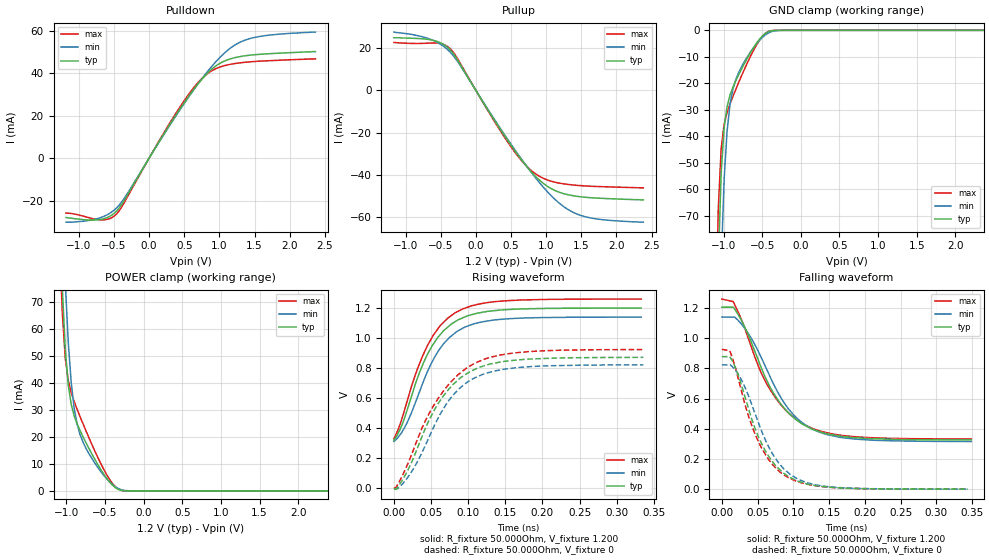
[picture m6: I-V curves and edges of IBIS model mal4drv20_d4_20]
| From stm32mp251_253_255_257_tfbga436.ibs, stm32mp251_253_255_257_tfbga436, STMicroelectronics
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[Model] mal4drv20_d4_20
Model_type   I/O
Polarity   Non-Inverting
Enable   Active-High
C_comp   1.838pF   1.835pF   1.848pF
C_comp_pullup   938.881fF   931.604fF   947.115fF
C_comp_pulldown 782.410fF   779.859fF   796.520fF
Vinh = 668.000mV
Vinl = 532.000mV
Vmeas = 600.000mV
Vref = 600.000mV
Rref = 50Ohms
Cref = 0pF
[Model Spec]
Vinh   668.000mV   638.000mV   698.000mV
Vinl   532.000mV   502.000mV   562.000mV
Vmeas   600.000mV   570.000mV   630.000mV
Vref   600.000mV   570.000mV   630.000mV
D_overshoot_ampl_h 0.24 NA   NA
D_overshoot_ampl_l 0.24 NA   NA
D_overshoot_area_l 300.000m NA   NA
D_overshoot_area_h 300.000m NA   NA
[Receiver Thresholds]
Vth = 600.000mV
Vth_min = 570.000mV
Vth_max = 630.000mV
Vinh_ac = 68.000mV
Vinh_dc = 68.000mV
Vinl_ac = -68.000mV
Vinl_dc = -68.000mV
Tslew_ac = 5.000ns
Threshold_sensitivity = 0.5
Reference_supply Pullup_ref
[Temperature Range]   25.000   125.000   -40.000
[Voltage Range]   1.200V   1.140V   1.260V
[GND Clamp Reference]   0.00V   0.00V   0.00V
[C Comp Corner]
| variable   typ   min   max
C_comp 1.848pF   1.838pF   1.835pF
C_comp_pullup 938.881fF   947.115fF   931.604fF
C_comp_pulldown 779.859fF   796.520fF   782.410fF
[Pulldown Reference]   0.00V   0.00V   0.00V
[POWER Clamp Reference]   1.200V   1.140V   1.260V
[Pullup Reference]   1.200V   1.140V   1.260V
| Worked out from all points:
|   slope of the pulldown table from 0 to 0.18 V, typ, clamps not added: 18.4 ohm
|   slope of the pullup table from 0 to 0.18 V, typ, clamps not added: 18.5 ohm
|   GND clamp passes 1 mA (typ) near -0.45 V on its own axis
|   POWER clamp passes 1 mA (typ) near -0.35 V on its own axis
|   rising waveform, R_fixture 50.000Ohm, V_fixture 1.200: 20-80 % time 46.3ps typ, 47.6ps min, 47ps max; typ from 0.321 V to 1.2 V
|   rising waveform, R_fixture 50.000Ohm, V_fixture 0: 20-80 % time 57.2ps typ, 56.6ps min, 62.2ps max; typ from -0.006 V to 0.872 V
|   falling waveform, R_fixture 50.000Ohm, V_fixture 1.200: 20-80 % time 57.7ps typ, 58.7ps min, 59.1ps max; typ from 1.21 V to 0.327 V
|   falling waveform, R_fixture 50.000Ohm, V_fixture 0: 20-80 % time 45.2ps typ, 47.2ps min, 44.8ps max; typ from 0.879 V to 0 V
[GND Clamp]
-1.184V   -365mA     -429.3mA   -336.5mA
-1.107V   -152.4mA   -215.7mA   -121.1mA
-1.069V   -88.87mA   -140.5mA   -67.62mA
-1.031V   -53.54mA   -88.39mA   -44.48mA
-992.7mV  -36.7mA    -56.18mA   -35.42mA
-954.6mV  -28.78mA   -37.93mA   -30.92mA
-916.4mV  -24.43mA   -27.89mA   -27.7mA
-840mV    -18.89mA   -18.42mA   -22.12mA
-763.6mV  -14.38mA   -13.51mA   -16.88mA
-572.7mV  -4.818mA   -5.067mA   -5.477mA
-458.2mV  -1.146mA   -1.695mA   -1.103mA
2.367V    25.44nA    625nA      8.401nA
[Power Clamp]
-1.167V   197.6mA    234.2mA    183.1mA
-1.091V   108mA      144mA      94.42mA
-1.053V   75.21mA    107.2mA    65.93mA
-1.015V   52.65mA    77.42mA    49.33mA
-976.4mV  39.37mA    55.31mA    41.02mA
-938.2mV  32.15mA    40.29mA    36.48mA
-900mV    27.91mA    30.75mA    33.22mA
-823.6mV  22.42mA    20.91mA    27.62mA
-632.7mV  11.76mA    10.36mA    14.83mA
-365.4mV  1.178mA    1.496mA    1.508mA
-212.7mV  14.35uA    76.22uA    9.056uA
2.384V    -16.74nA   -562.7nA   -5.86nA
[Pulldown]
-1.184V   -28mA      -30.2mA    -25.9mA
-725.5mV  -29.07mA   -28.41mA   -29mA
-572.7mV  -27.67mA   -26.26mA   -28.66mA
-458.2mV  -24.75mA   -23.28mA   -26.13mA
-343.6mV  -19.28mA   -18.42mA   -20.31mA
458.2mV   24.11mA    23.68mA    25.02mA
687.3mV   34.55mA    34.52mA    35.24mA
878.2mV   41.46mA    42.63mA    40.85mA
1.145V    46.59mA    51.48mA    44.06mA
1.375V    48.18mA    55.64mA    45.11mA
1.718V    49.14mA    57.9mA     45.84mA
2.367V    50.1mA     59.3mA     46.7mA
[Pullup]
-1.167V   25mA       27.69mA    22.76mA
-632.7mV  23.95mA    24.08mA    22.51mA
-480mV    22.2mA     21.43mA    22.03mA
-365.4mV  19.23mA    18.18mA    19.8mA
-289.1mV  15.9mA     15.07mA    16.58mA
474.6mV   -24.78mA   -24.26mA   -25.51mA
703.6mV   -35.24mA   -35.07mA   -35.28mA
894.5mV   -42.23mA   -43.31mA   -40.52mA
1.2V      -48.44mA   -53.83mA   -44.05mA
1.467V    -50.34mA   -58.99mA   -45.1mA
1.811V    -51.21mA   -61.33mA   -45.66mA
2.384V    -51.9mA    -62.5mA    -46.2mA
[Ramp]
R_load=50.000Ohm
dV/dt_r   523.800mV/53.000ps  494.249mV/53.000ps  555.600mV/55.500ps
dV/dt_f   523.800mV/52.500ps  494.249mV/54.500ps  555.600mV/53.000ps
[Rising waveform]
R_fixture=50.000Ohm
V_fixture=1.200
V_fixture_min=1.140
V_fixture_max=1.260
0s        320.6mV    311.7mV    331.7mV
8ps       389mV      354.2mV    421.9mV
17ps      507.4mV    428.7mV    568mV
31ps      724mV      598mV      786.1mV
45ps      890.5mV    775.4mV    948.2mV
61ps      1.015V     923mV      1.074V
83ps      1.111V     1.037V     1.17V
109ps     1.162V     1.097V     1.22V
150ps     1.189V     1.128V     1.248V
333ps     1.2V       1.14V      1.26V
[Rising waveform]
R_fixture=50.000Ohm
V_fixture=0
0s        -5.72mV    -2.683mV   -596.7uV
10ps      43.14mV    20.58mV    70.78mV
26ps      198.3mV    127.7mV    252.7mV
42ps      395.3mV    281.6mV    446.4mV
59ps      559.6mV    462.4mV    594.3mV
81ps      697.6mV    628.1mV    730mV
108ps     789.7mV    733.5mV    830.5mV
133ps     830.9mV    778.5mV    875.9mV
176ps     858.8mV    807.8mV    908.5mV
336ps     871.7mV    822mV      923.9mV
[Falling waveform]
R_fixture=50.000Ohm
V_fixture=1.200
V_fixture_min=1.140
V_fixture_max=1.260
0s        1.206V     1.141V     1.26V
16ps      1.206V     1.141V     1.243V
32ps      1.076V     1.067V     1.067V
50ps      867mV      923.8mV    827.6mV
67ps      680.6mV    750.6mV    663.6mV
92ps      511.5mV    539.9mV    510.8mV
115ps     425.2mV    431.5mV    428.4mV
139ps     376.9mV    373.5mV    382.7mV
179ps     344mV      335.2mV    350.7mV
349ps     326.6mV    315.7mV    332.4mV
[Falling waveform]
R_fixture=50.000Ohm
V_fixture=0
0s        878.6mV    823.6mV    927.2mV
11ps      878.6mV    823.6mV    916.7mV
17ps      828mV      799.8mV    836.1mV
37ps      537.6mV    623mV      488.2mV
56ps      297.3mV    380.6mV    269mV
73ps      169.2mV    217.7mV    152.5mV
94ps      81.5mV     104.4mV    74.22mV
117ps     37.18mV    46.02mV    34.97mV
153ps     12.04mV    14.29mV    11.5mV
344ps     108.7uV    200.2uV    85.94uV
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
